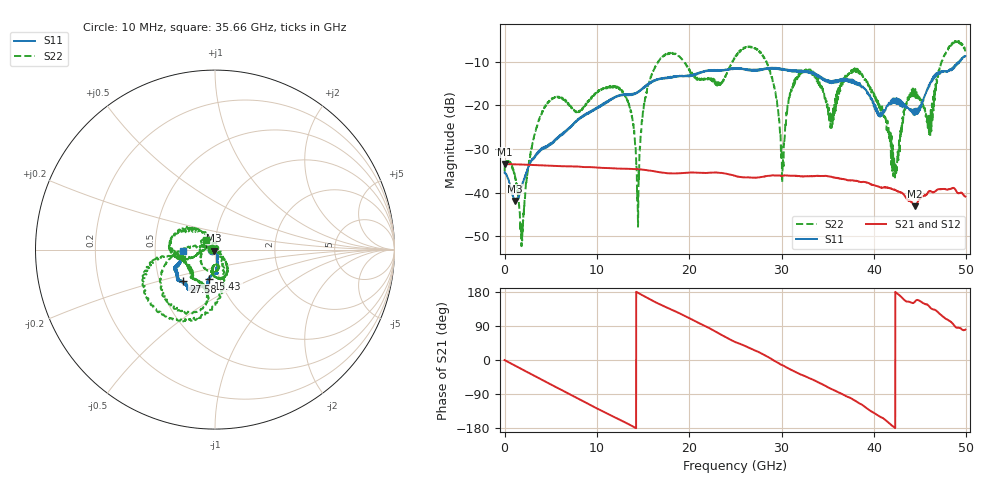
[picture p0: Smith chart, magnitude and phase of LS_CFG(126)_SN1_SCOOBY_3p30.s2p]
!Keysight Technologies,N5245B,MY58422026,A.13.80.08
!Date: Friday, March 20, 2020 00:06:48
!Correction: S11(Full 2 Port(1,2))
!S21(Full 2 Port(1,2))
!S12(Full 2 Port(1,2))
!S22(Full 2 Port(1,2))
!S2P File: Measurements: S11, S21, S12, S22:
# Hz S DB R 50.0
!freq dBS11 angS11 dBS21 angS21 dBS12 angS12 dBS22 angS22
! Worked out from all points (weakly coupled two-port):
!   4991 points, 10 MHz to 49.91 GHz, reference 50 ohm
!   highest |S21| = -33.42 dB at 10 MHz (marker M1); lowest = -43.1 dB at 44.42 GHz (marker M2)
!   lowest |S11| = -41.9 dB at 1.11 GHz (marker M3), VSWR 1.02, Z = 49.4 - j0.503 ohm
!   |S11| at or under -10 dB: start of sweep to 49.23 GHz; 49.30562 GHz to 49.32566 GHz (20.04 MHz wide, 0.0406 % of centre)
!   |S22| runs from -52.3 to -5.1 dB; largest |S21 - S12| = 0.00021
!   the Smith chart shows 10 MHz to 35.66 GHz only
!   S11 on the Smith chart (normalised r, x): 10 MHz: 0.97, -0.01; 15.43 GHz: 0.89, -0.30; 27.58 GHz: 0.66, -0.25; 35.66 GHz: 0.69, -0.01
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1e7  -35.38 -170.4  -33.42 -0.3  -33.37 -0.2  -35.09 177.0
1.11e9  -41.93 -140.5  -33.51 -14.5  -33.50 -14.5  -36.30 -116.0
1.87e9  -38.49 -75.2  -33.55 -24.3  -33.54 -24.2  -49.61 -5.1
4.22e9  -29.95 -58.5  -33.76 -54.3  -33.76 -54.3  -20.85 -151.4
8.33e9  -22.82 -79.6  -34.08 -107.0  -34.07 -106.9  -21.01 -93.0
1.276e10  -17.63 -84.2  -34.51 -161.0  -34.51 -161.0  -16.78 -63.1
1.445e10  -17.01 -96.0  -34.64 177.5  -34.62 177.5  -47.11 -115.3
1.543e10  -15.48 -101.9  -34.87 164.4  -34.86 164.5  -16.55 173.4
1.665e10  -14.04 -101.5  -35.27 148.9  -35.26 148.9  -9.98 -157.4
2.496e10  -11.60 -124.7  -36.13 47.7  -36.11 47.8  -9.08 -167.9
2.758e10  -12.02 -134.9  -36.51 20.3  -36.49 20.4  -7.68 -110.1
3.011e10  -11.86 -143.7  -36.14 -13.5  -36.14 -13.4  -34.66 15.9
3.116e10  -12.02 -148.4  -36.14 -27.3  -36.14 -27.1  -15.59 140.1
3.328e10  -12.51 -157.9  -36.21 -51.0  -36.23 -50.8  -12.32 -175.3
3.566e10  -14.81 -178.1  -36.49 -79.5  -36.43 -79.2  -21.97 129.8
3.816e10  -15.26 174.8  -37.34 -110.5  -37.28 -110.8  -11.58 -174.7
4.16e10  -19.53 105.6  -38.93 -165.6  -38.93 -166.0  -25.65 67.5
4.233e10  -18.67 105.3  -39.42 179.6  -39.43 179.5  -33.75 164.8
4.442e10  -22.24 57.7  -43.14 153.6  -43.14 153.8  -17.79 -11.2
4.601e10  -15.57 6.6  -39.63 140.9  -39.64 140.8  -23.30 116.9
4.771e10  -12.18 6.9  -39.17 110.0  -39.20 109.8  -8.16 -80.0
4.991e10  -8.69 -12.8  -40.90 80.1  -40.92 79.7  -7.37 -14.8
